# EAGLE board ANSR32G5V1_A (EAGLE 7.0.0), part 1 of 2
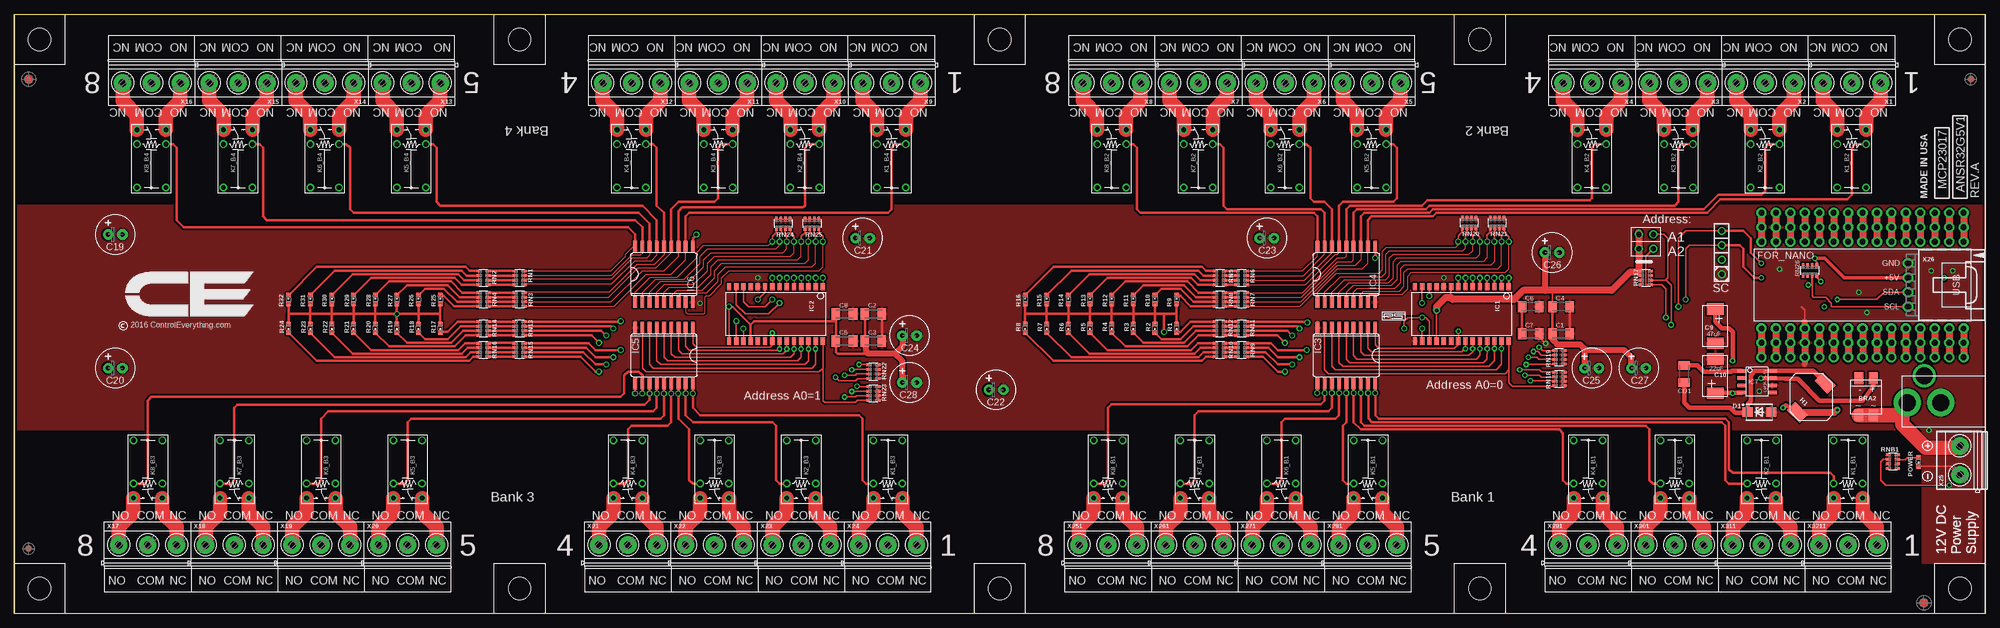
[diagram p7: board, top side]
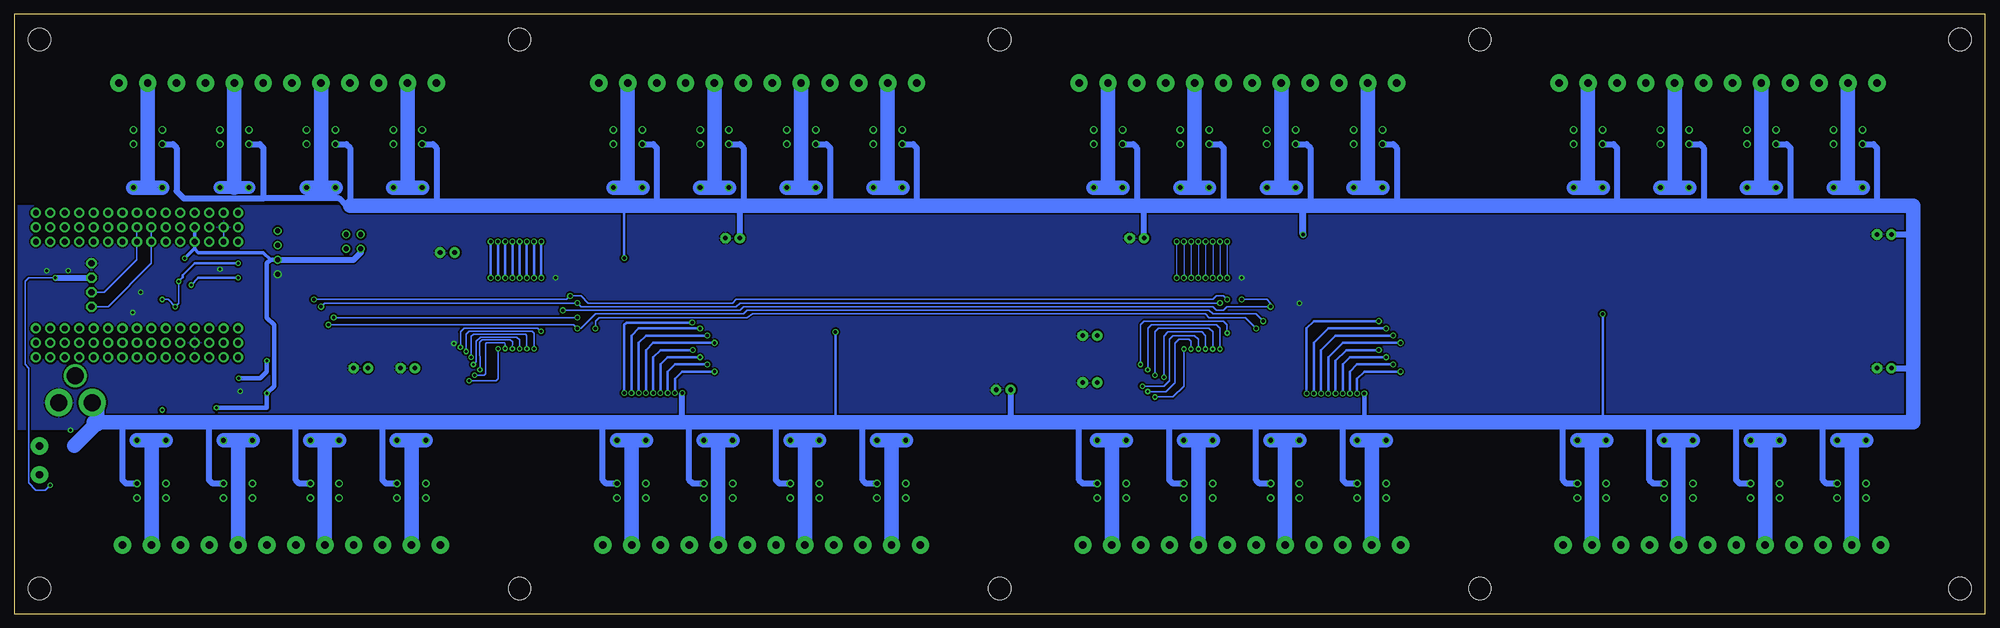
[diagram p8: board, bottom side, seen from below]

Size 346.71 x 105.42 mm. Coordinates in mm from the lower left corner, seen from the top.
Outline: 346.71,71.77 346.71,13.98
Outline: 0,105.42 346.69,105.42 346.69,0 0,0 0,105.42
Copper layers (1*16): Top 0.035mm / dielectric 1.5mm / Bottom 0.035mm
Design rules "default *": minimum track width 6mil, minimum drill 12mil, track to track 5mil, track to pad 5mil, pad to pad 5mil, via to via 5mil, smd to smd 5mil, copper to edge 20mil, drill to drill 8mil, minimum pad ring 10mil, minimum via ring 8mil, stop-mask expansion 4mil, vias tented up to drill 0mil, thermal gap 10mil

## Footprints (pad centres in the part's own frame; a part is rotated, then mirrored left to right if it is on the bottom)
MB2S = smd 1.55 x 2.1: + 0,-6.5; - 2.54,-6.5; ~@1 0,0; ~@2 2.54,0
_CA_.1UF_50V = smd 1.5 x 2: 1 -1.5,0; 2 1.5,0
_CB_10UF_25V = smd 1.5 x 2: 1 -1.5,0; 2 1.5,0
C2917(7343)-Y = smd 2 x 3: 1 -3,0; 2 3,0
E-025X060 = drill 0.813 pad 1.778: + -1.27,0 | drill 0.813 pad 1.778 octagon: - 1.27,0
_CD_10NF_50V = smd 1.5 x 2: 1 -1.5,0; 2 1.5,0
DO214AC_ZENER = smd 1.8 x 1.7: A 2.05,0; C -2.05,0
ARDUINO_NANO = drill 1 pad 1.778: 3V1 -2.54,-2.54; 3V3 0,-2.54; 5V 0,-27.94; 5V1 -2.54,-27.94; A0 0,-7.62; A1 0,-10.16; A2 0,-12.7; A3 0,-15.24; A4 0,-17.78; A5 0,-20.32; A6 0,-22.86; A7 0,-25.4; A8 -2.54,-7.62; A9 -2.54,-10.16; A10 -2.54,-12.7; A11 -2.54,-15.24; A12 -2.54,-17.78; A13 -2.54,-20.32; A14 -2.54,-22.86; A15 -2.54,-25.4; D1 -2.54,0; D2 20.32,-25.4; D3 20.32,-22.86; D4 20.32,-20.32; D5 20.32,-17.78; D6 20.32,-15.24; D7 20.32,-12.7; D8 20.32,-10.16; D9 20.32,-7.62; D10 20.32,-5.08; D11 20.32,-2.54; D12 20.32,0; D13 0,0; D14 22.86,0; D15 22.86,-2.54; D16 22.86,-5.08; D17 22.86,-7.62; D18 22.86,-10.16; D19 22.86,-12.7; D20 22.86,-15.24; D21 22.86,-17.78; D22 22.86,-20.32; D23 22.86,-22.86; D24 22.86,-25.4; GND 0,-33.02; GND1 -2.54,-33.02; GND@1 20.32,-27.94; GND@2 22.86,-27.94; P$16 2.54,0; P$17 2.54,-2.54; P$18 2.54,-5.08; P$19 2.54,-7.62; P$20 2.54,-10.16; P$21 2.54,-12.7; P$22 2.54,-15.24; P$23 2.54,-17.78; P$24 2.54,-20.32; P$25 2.54,-22.86; P$26 2.54,-25.4; P$27 2.54,-27.94; P$28 2.54,-30.48; P$29 2.54,-33.02; P$30 2.54,-35.56; P$31 17.78,0; P$32 17.78,-2.54; P$33 17.78,-5.08; P$34 17.78,-7.62; P$35 17.78,-10.16; P$36 17.78,-12.7; P$37 17.78,-15.24; P$38 17.78,-17.78; P$39 17.78,-20.32; P$40 17.78,-22.86; P$41 17.78,-25.4; P$42 17.78,-27.94; P$43 17.78,-30.48; P$44 17.78,-33.02; P$45 17.78,-35.56; REF 0,-5.08; REF1 -2.54,-5.08; RST 0,-30.48; RST1 -2.54,-30.48; RST@1 20.32,-30.48; RST@2 22.86,-30.48; RX0 20.32,-33.02; RX1 22.86,-33.02; TX1 20.32,-35.56; TX2 22.86,-35.56; VIN 0,-35.56; VIN1 -2.54,-35.56
IND_ELL8TP = smd 2.054 x 3.2 rotated 45: 1 -2.442,-2.696; 2 2.442,2.442
SO28W = smd 0.762 x 1.27: 1 -7.62,-4.78; 2 -6.35,-4.78; 3 -5.08,-4.78; 4 -3.81,-4.78; 5 -2.54,-4.78; 6 -1.27,-4.78; 7 0,-4.78; 8 1.27,-4.78; 9 2.54,-4.78; 10 3.81,-4.78; 11 5.08,-4.78; 12 6.35,-4.78; 13 7.62,-4.78; 14 8.89,-4.78; 15 8.89,4.78; 16 7.62,4.78; 17 6.35,4.78; 18 5.08,4.78; 19 3.81,4.78; 20 2.54,4.78; 21 1.27,4.78; 22 0,4.78; 23 -1.27,4.78; 24 -2.54,4.78; 25 -3.81,4.78; 26 -5.08,4.78; 27 -6.35,4.78; 28 -7.62,4.78
SO18L = smd 0.66 x 2.032: 1 -5.08,-4.902; 2 -3.81,-4.902; 3 -2.54,-4.902; 4 -1.27,-4.902; 5 0,-4.902; 6 1.27,-4.902; 7 2.54,-4.902; 8 3.81,-4.902; 9 5.08,-4.902; 10 5.08,4.902; 11 3.81,4.902; 12 2.54,4.902; 13 1.27,4.902; 14 0,4.902; 15 -1.27,4.902; 16 -2.54,4.902; 17 -3.81,4.902; 18 -5.08,4.902
SO-8 = smd 0.6 x 1.55: 1 -1.905,-2.69; 2 -0.635,-2.69; 3 0.635,-2.69; 4 1.905,-2.69; 5 1.905,2.71; 6 0.635,2.71; 7 -0.635,2.71; 8 -1.905,2.71
G5V1 = drill 0.813: C1 -2.54,2.54; C2 -2.54,-2.54; COM@1 5.08,-2.54; COM@2 5.08,2.54; NC -5.08,-2.54; NO -5.08,2.54
CHIPLED_0603 = smd 0.8 x 0.8: A 0,-0.75; C 0,0.75
RNB = smd 0.5 x 0.9: 1 -1.2,-0.8; 2 -0.4,-0.8; 3 0.4,-0.8; 4 1.2,-0.8; 5 1.2,0.8; 6 0.4,0.8; 7 -0.4,0.8; 8 -1.2,0.8
RNE = smd 0.5 x 0.9: 1 -1.2,-0.8; 2 -0.4,-0.8; 3 0.4,-0.8; 4 1.2,-0.8; 5 1.2,0.8; 6 0.4,0.8; 7 -0.4,0.8; 8 -1.2,0.8
RND = smd 0.5 x 0.9: 1 -1.2,-0.8; 2 -0.4,-0.8; 3 0.4,-0.8; 4 1.2,-0.8; 5 1.2,0.8; 6 0.4,0.8; 7 -0.4,0.8; 8 -1.2,0.8
PCB_MOUNTING_HOLE = hole 3.962: 4.445,4.445
JUMPER_2X2 = drill 0.9: A1 0,2.54; A2 0,0; B1 2.54,2.54; B2 2.54,0
PJ-102A = drill 3 pad 4.8: RING 0.1,-3.39; TIP 0.1,-9.29 | drill 3 pad 3.251: RING_SW -4.6,-6.29
MKDSN1,5/3-5,08 = drill 1.3 pad 3.048: 1 -7.641,0.025; 2 -2.561,0.025; 3 2.519,0.025
MKDSN1,5/2-5,08 = drill 1.3 pad 3.048: 1 -2.561,0.025; 2 2.519,0.025
70553-04 = drill 1.1 pad 1.778 octagon: 1 -3.81,-7.62; 2 -1.27,-7.62; 3 1.27,-7.62; 4 3.81,-7.62

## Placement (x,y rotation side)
BRA2  MB2S_  [MB2S]  327.02,34.94 180 top
C1  [_CA_.1UF_50V]  272.1,49.22 0 top
C2  _CB_10UF_25VC1206K  [_CB_10UF_25V]  151.13,52.72 0 top
C3  [_CA_.1UF_50V]  151.13,47.95 0 top
C4  _CB_10UF_25VC1206K  [_CB_10UF_25V]  272.1,53.99 0 top
C5  [_CA_.1UF_50V]  146.05,47.95 0 top
C6  _CB_10UF_25VC1206K  [_CB_10UF_25V]  266.7,53.99 0 top
C7  [_CA_.1UF_50V]  266.7,49.22 0 top
C8  _CB_10UF_25VC1206K  [_CB_10UF_25V]  146.05,52.72 0 top
C9  47uF  [C2917(7343)-Y]  299.21,50.56 270 top
C10  22uF  [C2917(7343)-Y]  299.21,41.77 90 top
C19  100uF  [E-025X060]  17.78,66.69 0 top
C20  100uF  [E-025X060]  17.78,43.19 0 top
C21  100uF  [E-025X060]  149.22,66.05 0 top
C22  100uF  [E-025X060]  172.72,39.38 0 top
C23  100uF  [E-025X060]  220.34,66.05 0 top
C24  100uF  [E-025X060]  157.48,48.91 0 top
C25  100uF  [E-025X060]  277.5,43.19 0 top
C26  100uF  [E-025X060]  270.51,63.51 0 top
C27  100uF  [E-025X060]  285.75,43.19 0 top
C28  100uF  [E-025X060]  157.48,40.65 0 top
CD1  [_CD_10NF_50V]  293.75,42.18 270 top
D1  B360A  [DO214AC_ZENER]  306.96,35.45 0 top
FOR_NANO  ARDUINO_NANO  [ARDUINO_NANO]  342.9,67.96 270 top
H1  ELL8TP  [IND_ELL8TP]  316.1,38.11 0 top
IC1  MCP23017SO  [SO28W]  255.27,52.72 180 top
IC2  MCP23017SO  [SO28W]  134.62,52.72 180 top
IC3  ULN2803  [SO18L]  234.31,45.42 180 top
IC4  ULN2803  [SO18L]  234.31,59.7 0 top
IC5  ULN2803  [SO18L]  114.3,45.42 180 top
IC6  ULN2803  [SO18L]  114.3,59.7 0 top
IC7  LM2675-5V  [SO-8]  306.58,40.78 270 top
K1_B1  G5V1  [G5V1]  322.58,25.41 90 top
K1_B2  G5V1  [G5V1]  323.21,80.02 270 top
K1_B3  G5V1  [G5V1]  153.67,25.41 90 top
K1_B4  G5V1  [G5V1]  154.31,80.02 270 top
K2_B1  G5V1  [G5V1]  307.34,25.41 90 top
K2_B2  G5V1  [G5V1]  307.98,80.02 270 top
K2_B3  G5V1  [G5V1]  138.43,25.41 90 top
K2_B4  G5V1  [G5V1]  139.06,80.02 270 top
K3_B1  G5V1  [G5V1]  292.1,25.41 90 top
K3_B2  G5V1  [G5V1]  292.74,80.02 270 top
K3_B3  G5V1  [G5V1]  123.19,25.41 90 top
K3_B4  G5V1  [G5V1]  123.83,80.02 270 top
K4_B1  G5V1  [G5V1]  276.86,25.41 90 top
K4_B2  G5V1  [G5V1]  277.5,80.02 270 top
K4_B3  G5V1  [G5V1]  107.95,25.41 90 top
K4_B4  G5V1  [G5V1]  108.58,80.02 270 top
K5_B1  G5V1  [G5V1]  238.12,25.41 90 top
K5_B2  G5V1  [G5V1]  238.76,80.02 270 top
K5_B3  G5V1  [G5V1]  69.22,25.41 90 top
K5_B4  G5V1  [G5V1]  69.85,80.02 270 top
K6_B1  G5V1  [G5V1]  222.88,25.41 90 top
K6_B2  G5V1  [G5V1]  223.52,80.02 270 top
K6_B3  G5V1  [G5V1]  53.98,25.41 90 top
K6_B4  G5V1  [G5V1]  54.61,80.02 270 top
K7_B1  G5V1  [G5V1]  207.65,25.41 90 top
K7_B2  G5V1  [G5V1]  208.28,80.02 270 top
K7_B3  G5V1  [G5V1]  38.73,25.41 90 top
K7_B4  G5V1  [G5V1]  39.37,80.02 270 top
K8_B1  G5V1  [G5V1]  192.41,25.41 90 top
K8_B2  G5V1  [G5V1]  193.04,80.02 270 top
K8_B3  G5V1  [G5V1]  23.5,25.41 90 top
K8_B4  G5V1  [G5V1]  24.13,80.02 270 top
POWER  LED_NCD  [CHIPLED_0603]  334.96,26.68 180 top
R1  LED_NCD  [CHIPLED_0603]  204.47,50.18 180 top
R2  LED_NCD  [CHIPLED_0603]  200.66,50.18 180 top
R3  LED_NCD  [CHIPLED_0603]  196.85,50.18 180 top
R4  LED_NCD  [CHIPLED_0603]  193.04,50.18 180 top
R5  LED_NCD  [CHIPLED_0603]  189.23,50.18 180 top
R6  LED_NCD  [CHIPLED_0603]  185.42,50.18 180 top
R7  LED_NCD  [CHIPLED_0603]  181.61,50.18 180 top
R8  LED_NCD  [CHIPLED_0603]  177.8,50.18 180 top
R9  LED_NCD  [CHIPLED_0603]  204.47,55.26 0 top
R10  LED_NCD  [CHIPLED_0603]  200.66,55.26 0 top
R11  LED_NCD  [CHIPLED_0603]  196.85,55.26 0 top
R12  LED_NCD  [CHIPLED_0603]  193.04,55.26 0 top
R13  LED_NCD  [CHIPLED_0603]  189.23,55.26 0 top
R14  LED_NCD  [CHIPLED_0603]  185.42,55.26 0 top
R15  LED_NCD  [CHIPLED_0603]  181.61,55.26 0 top
R16  LED_NCD  [CHIPLED_0603]  177.8,55.26 0 top
R17  LED_NCD  [CHIPLED_0603]  74.93,50.18 180 top
R18  LED_NCD  [CHIPLED_0603]  71.12,50.18 180 top
R19  LED_NCD  [CHIPLED_0603]  67.31,50.18 180 top
R20  LED_NCD  [CHIPLED_0603]  63.5,50.18 180 top
R21  LED_NCD  [CHIPLED_0603]  59.69,50.18 180 top
R22  LED_NCD  [CHIPLED_0603]  55.88,50.18 180 top
R23  LED_NCD  [CHIPLED_0603]  52.07,50.18 180 top
R24  LED_NCD  [CHIPLED_0603]  48.26,50.18 180 top
R25  LED_NCD  [CHIPLED_0603]  74.93,55.26 0 top
R26  LED_NCD  [CHIPLED_0603]  71.12,55.26 0 top
R27  LED_NCD  [CHIPLED_0603]  67.31,55.26 0 top
R28  LED_NCD  [CHIPLED_0603]  63.5,55.26 0 top
R29  LED_NCD  [CHIPLED_0603]  59.69,55.26 0 top
R30  LED_NCD  [CHIPLED_0603]  55.88,55.26 0 top
R31  LED_NCD  [CHIPLED_0603]  52.07,55.26 0 top
R32  LED_NCD  [CHIPLED_0603]  48.26,55.26 0 top
RN1  _RNB_510  [RNB]  88.9,59.07 90 top
RN2  _RNB_510  [RNB]  82.55,59.07 90 top
RN3  _RNB_510  [RNB]  88.9,55.26 270 top
RN4  _RNB_510  [RNB]  82.55,55.26 270 top
RN5  _RNB_510  [RNB]  212.09,59.07 270 top
RN6  _RNB_510  [RNB]  215.9,59.07 270 top
RN7  _RNB_510  [RNB]  215.9,55.26 270 top
RN8  _RNB_510  [RNB]  212.09,55.26 270 top
RN9  _RNB_510  [RNB]  215.9,46.37 270 top
RN10  _RNB_510  [RNB]  212.09,46.37 270 top
RN11  _RNB_510  [RNB]  215.9,50.18 90 top
RN12  _RNB_510  [RNB]  212.09,50.18 90 top
RN13  _RNB_510  [RNB]  88.9,50.18 270 top
RN14  _RNB_510  [RNB]  82.55,50.18 270 top
RN15  _RNB_510  [RNB]  88.9,46.37 270 top
RN16  _RNB_510  [RNB]  82.55,46.37 270 top
RN17  _RNE_10K  [RNE]  287.02,59.07 270 top
RN18  _RNE_10K  [RNE]  271.78,41.29 90 top
RN19  _RNE_10K  [RNE]  271.78,45.1 90 top
RN20  _RNE_10K  [RNE]  255.91,68.72 180 top
RN21  _RNE_10K  [RNE]  260.86,68.72 180 top
RN22  _RNE_10K  [RNE]  151.13,42.56 90 top
RN23  _RNE_10K  [RNE]  151.13,38.75 90 top
RN24  _RNE_10K  [RNE]  135.25,68.59 180 top
RN25  _RNE_10K  [RNE]  140.34,68.59 180 top
RN26  _RND_4.7K  [RND]  315.85,60.34 0 top
RNB1  _RNB_510  [RNB]  330.45,26.75 90 top
U$1  PCB_MOUNTING_HOLE  [PCB_MOUNTING_HOLE]  262.25,96.53 90 top
U$2  PCB_MOUNTING_HOLE  [PCB_MOUNTING_HOLE]  177.8,96.53 90 top
U$3  PCB_MOUNTING_HOLE  [PCB_MOUNTING_HOLE]  346.71,96.53 90 top
U$4  PCB_MOUNTING_HOLE  [PCB_MOUNTING_HOLE]  84.45,8.9 270 top
U$5  PCB_MOUNTING_HOLE  [PCB_MOUNTING_HOLE]  168.91,8.9 270 top
U$6  PCB_MOUNTING_HOLE  [PCB_MOUNTING_HOLE]  0,8.9 270 top
U$7  PCB_MOUNTING_HOLE  [PCB_MOUNTING_HOLE]  93.34,96.53 90 top
U$8  PCB_MOUNTING_HOLE  [PCB_MOUNTING_HOLE]  8.89,96.53 90 top
U$9  PCB_MOUNTING_HOLE  [PCB_MOUNTING_HOLE]  177.8,96.53 90 top
U$10  PCB_MOUNTING_HOLE  [PCB_MOUNTING_HOLE]  253.37,8.9 270 top
U$11  PCB_MOUNTING_HOLE  [PCB_MOUNTING_HOLE]  337.82,8.9 270 top
U$12  PCB_MOUNTING_HOLE  [PCB_MOUNTING_HOLE]  168.91,8.9 270 top
U$13  JUMPER_2X2  [JUMPER_2X2]  285.75,66.69 270 top
U$14  2.1MMJACK  [PJ-102A]  342.26,37.22 270 top
U$15  [VISION_REF15]  335.92,1.92 90 top
U$18  [VISION_REF10]  344.17,93.99 90 top
U$19  [ICON_MINUS]  336.55,24.14 90 top
U$20  [ICON_PLUS]  336.55,29.54 0 top
U$21  [ICON_USA]  336.55,73.04 90 top
U$22  [ICON_MINUS]  336.55,24.14 90 top
U$23  [VISION_REF15]  2.54,93.99 90 top
U$24  [ICON_PLUS]  336.55,29.54 0 top
U$26  [ICON_MINUS]  336.55,24.14 90 top
U$27  [ICON_PLUS]  336.55,29.54 0 top
U$28  [VISION_REF10]  2.54,11.44 90 top
X1  MKDSN1,5/3-5,08  [MKDSN1,5/3-5,08]  320.68,93.36 180 top
X2  MKDSN1,5/3-5,08  [MKDSN1,5/3-5,08]  305.44,93.36 180 top
X3  MKDSN1,5/3-5,08  [MKDSN1,5/3-5,08]  290.19,93.36 180 top
X4  MKDSN1,5/3-5,08  [MKDSN1,5/3-5,08]  274.95,93.36 180 top
X5  MKDSN1,5/3-5,08  [MKDSN1,5/3-5,08]  236.22,93.36 180 top
X6  MKDSN1,5/3-5,08  [MKDSN1,5/3-5,08]  220.98,93.36 180 top
X7  MKDSN1,5/3-5,08  [MKDSN1,5/3-5,08]  205.74,93.36 180 top
X8  MKDSN1,5/3-5,08  [MKDSN1,5/3-5,08]  190.5,93.36 180 top
X9  MKDSN1,5/3-5,08  [MKDSN1,5/3-5,08]  151.76,93.36 180 top
X10  MKDSN1,5/3-5,08  [MKDSN1,5/3-5,08]  136.53,93.36 180 top
X11  MKDSN1,5/3-5,08  [MKDSN1,5/3-5,08]  121.28,93.36 180 top
X12  MKDSN1,5/3-5,08  [MKDSN1,5/3-5,08]  106.05,93.36 180 top
X13  MKDSN1,5/3-5,08  [MKDSN1,5/3-5,08]  67.31,93.36 180 top
X14  MKDSN1,5/3-5,08  [MKDSN1,5/3-5,08]  52.07,93.36 180 top
X15  MKDSN1,5/3-5,08  [MKDSN1,5/3-5,08]  36.83,93.36 180 top
X16  MKDSN1,5/3-5,08  [MKDSN1,5/3-5,08]  21.59,93.36 180 top
X17  MKDSN1,5/3-5,08  [MKDSN1,5/3-5,08]  26.04,12.08 0 top
X18  MKDSN1,5/3-5,08  [MKDSN1,5/3-5,08]  41.27,12.08 0 top
X19  MKDSN1,5/3-5,08  [MKDSN1,5/3-5,08]  56.52,12.08 0 top
X20  MKDSN1,5/3-5,08  [MKDSN1,5/3-5,08]  71.75,12.08 0 top
X21  MKDSN1,5/3-5,08  [MKDSN1,5/3-5,08]  110.49,12.08 0 top
X22  MKDSN1,5/3-5,08  [MKDSN1,5/3-5,08]  125.73,12.08 0 top
X23  MKDSN1,5/3-5,08  [MKDSN1,5/3-5,08]  140.97,12.08 0 top
X24  MKDSN1,5/3-5,08  [MKDSN1,5/3-5,08]  156.21,12.08 0 top
X25  MKDSN1,5/2-5,08  [MKDSN1,5/2-5,08]  342.26,27 90 top
X26  C-GRID-04-70553  [70553-04]  340.74,57.8 270 top
X251  MKDSN1,5/3-5,08  [MKDSN1,5/3-5,08]  194.94,12.08 0 top
X261  MKDSN1,5/3-5,08  [MKDSN1,5/3-5,08]  210.19,12.08 0 top
X271  MKDSN1,5/3-5,08  [MKDSN1,5/3-5,08]  225.43,12.08 0 top
X281  MKDSN1,5/3-5,08  [MKDSN1,5/3-5,08]  240.66,12.08 0 top
X291  MKDSN1,5/3-5,08  [MKDSN1,5/3-5,08]  279.4,12.08 0 top
X301  MKDSN1,5/3-5,08  [MKDSN1,5/3-5,08]  294.64,12.08 0 top
X311  MKDSN1,5/3-5,08  [MKDSN1,5/3-5,08]  309.88,12.08 0 top
X3211  MKDSN1,5/3-5,08  [MKDSN1,5/3-5,08]  325.12,12.08 0 top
